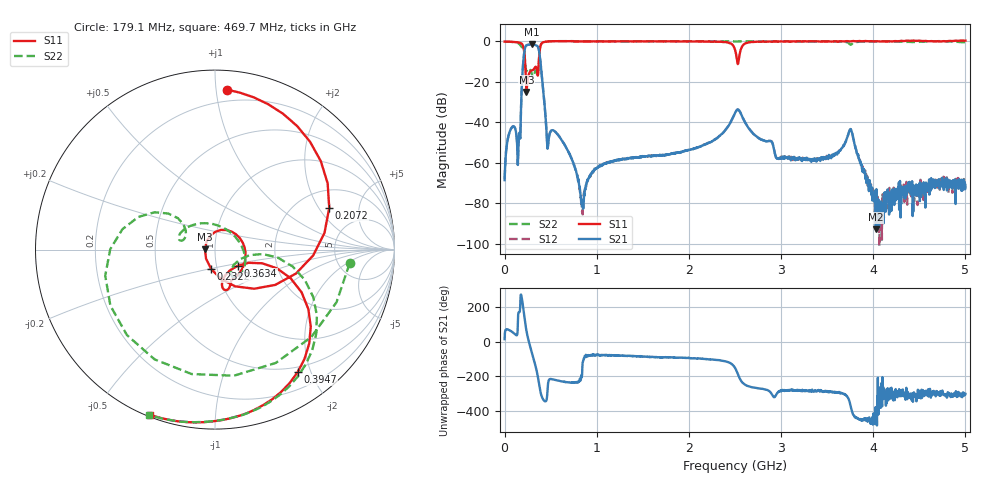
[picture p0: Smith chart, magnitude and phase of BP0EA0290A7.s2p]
!Agilent Technologies,E8358A,US41080443,A.07.50.56
!Agilent E8358A: A.07.50.56
!Date: Friday, November 10, 2017 09:08:13
!Correction: S11(Full 2 Port(1,2))
!S21(Full 2 Port(1,2))
!S12(Full 2 Port(1,2))
!S22(Full 2 Port(1,2))
!S2P File: Measurements: S11, S21, S12, S22:
# Hz S  dB  R 50
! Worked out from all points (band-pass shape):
!   1601 points, 1 MHz to 5 GHz, reference 50 ohm
!   highest |S21| = -1.58 dB at 297.8 MHz (marker M1); lowest = -92.9 dB at 4.028 GHz (marker M2)
!   |S21| within 3 dB of the highest: 217.1 MHz to 374.4 MHz (157.3 MHz wide, 53.2 % of centre)
!   lowest |S11| = -25.0 dB at 238.5 MHz (marker M3), VSWR 1.12, Z = 44.7 + j0.164 ohm
!   |S11| at or under -10 dB: 222.5 MHz to 371.3 MHz (148.8 MHz wide, 50.1 % of centre); 2.524 GHz to 2.539 GHz (14.49 MHz wide, 0.572 % of centre)
!   |S22| runs from -17.8 to 0.1 dB; largest |S21 - S12| = 0.0055
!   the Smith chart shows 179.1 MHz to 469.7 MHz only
!   S11 on the Smith chart (normalised r, x): 179.1 MHz: 0.12, +1.07; 207.2 MHz: 2.91, +2.50; 232.2 MHz: 0.94, -0.21; 363.4 MHz: 1.27, -0.23; 394.7 MHz: 0.43, -1.81; 469.7 MHz: 0.01, -0.68
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1000000  -0.15 179.7  -68.64 15.2  -67.95 16.5  -0.15 179.7
6.661188e7  -0.26 159.5  -43.61 62.9  -43.48 63.4  -0.27 156.6
1.384725e8  -0.50 126.0  -52.69 42.7  -52.63 43.0  -0.76 107.1
1.790894e8  -0.98 85.9  -33.19 -85.8  -33.13 -85.8  -2.45 -5.9
2.072088e8  -3.38 20.0  -8.26 179.2  -8.20 179.2  -4.03 -166.7
2.322038e8  -19.13 -101.1  -2.29 81.6  -2.23 81.6  -14.21 146.6
2.384525e8  -25.00 178.1  -2.02 62.3  -1.96 62.3  -14.90 159.4
2.978156e8  -14.38 -53.1  -1.58 -65.1  -1.54 -65.1  -16.47 103.4
3.634275e8  -16.18 -35.4  -2.79 151.9  -2.74 151.9  -16.53 -21.2
3.946712e8  -1.69 -55.9  -12.37 58.7  -12.33 58.7  -1.77 -51.7
4.696562e8  -0.10 -111.4  -52.45 103.1  -52.42 103.7  -0.09 -111.7
6.696162e8  0.06 -145.6  -52.67 126.2  -52.53 126.2  0.05 -146.0
8.352081e8  -0.05 -156.0  -80.22 167.2  -79.24 167.1  -0.09 -156.3
1.669416e9  -0.07 -175.8  -56.44 -90.2  -56.35 -89.5  -0.08 -175.8
2.369276e9  -0.38 159.9  -45.35 -110.2  -45.29 -110.3  -0.10 173.2
2.5005e9  -4.15 101.9  -35.52 -151.0  -35.52 -151.3  -0.10 170.9
2.578609e9  -2.50 -127.0  -37.22 124.7  -37.23 125.1  -0.14 169.8
3.334708e9  -0.02 168.6  -58.24 76.7  -58.70 75.5  -0.08 158.0
3.753374e9  -0.04 160.9  -43.37 -8.8  -43.39 -9.5  -1.70 152.7
4.028319e9  -0.02 156.2  -92.89 -76.0  -77.36 -71.7  -0.10 152.8
4.168916e9  0.01 153.4  -77.45 71.2  -73.63 44.9  -0.04 152.2
5e9  0.31 144.1  -71.00 57.9  -71.43 41.3  -0.48 151.6
